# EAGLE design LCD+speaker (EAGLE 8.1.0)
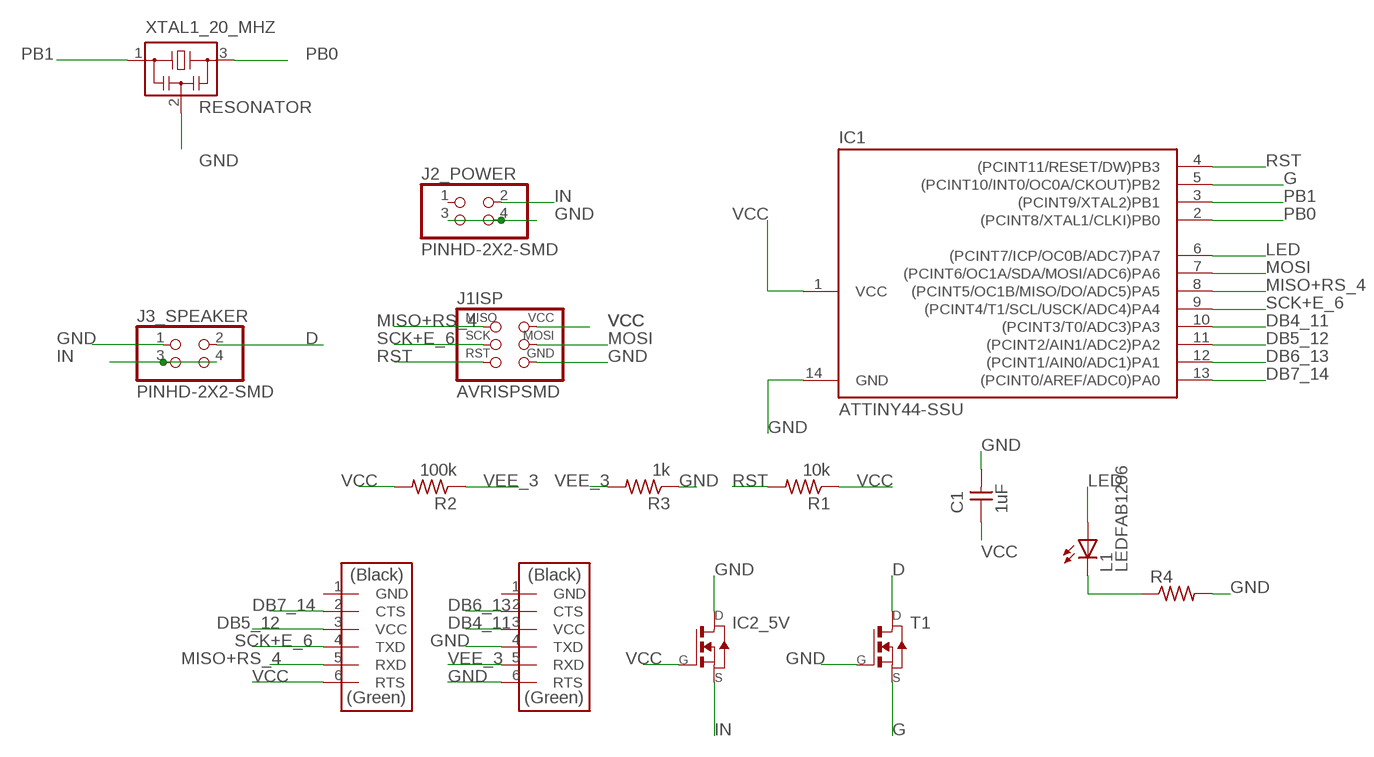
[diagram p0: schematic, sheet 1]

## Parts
C1  1uF  CAP-UNPOLARIZED  [C1206]
IC1  ATTINY44-SSU  [SOIC14]
IC2_5V  NMOSFETSOT23  [SOT-23]
J1ISP  AVRISPSMD  [2X03SMD]
J2_POWER  PINHD-2X2-SMD  [2X02SMD]
J3_SPEAKER  PINHD-2X2-SMD  [2X02SMD]
L1  LEDFAB1206  [LED1206FAB]
R1  10k  RES-US1206FAB  [R1206FAB]
R2  100k  RES-US1206FAB  [R1206FAB]
R3  1k  RES-US1206FAB  [R1206FAB]
R4  RES-US1206FAB  [R1206FAB]
T1  NMOSFETSOT23  [SOT-23]
U$1  FTDI-SMD-HEADER  [1X06SMD]
U$2  FTDI-SMD-HEADER  [1X06SMD]
XTAL1_20_MHZ  RESONATOR  [EFOBM]

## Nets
D: J3_SPEAKER.2 T1.1(D)
DB4_11: IC1.10((PCINT3/T0/ADC3)PA3) U$2.3(VCC)
DB5_12: IC1.11((PCINT2/AIN1/ADC2)PA2) U$1.3(VCC)
DB6_13: IC1.12((PCINT1/AIN0/ADC1)PA1) U$2.2(CTS)
DB7_14: IC1.13((PCINT0/AREF/ADC0)PA0) U$1.2(CTS)
G: IC1.5((PCINT10/INT0/OC0A/CKOUT)PB2) T1.2(S)
GND: C1.2 IC1.14(GND) IC2_5V.1(D) J1ISP.6(GND) J2_POWER.3 J2_POWER.4 J3_SPEAKER.1 R3.1 R4.2 T1.3(G) U$2.4(TXD) U$2.6(RTS) XTAL1_20_MHZ.2
IN: IC2_5V.2(S) J2_POWER.2 J3_SPEAKER.3 J3_SPEAKER.4
LED: IC1.6((PCINT7/ICP/OC0B/ADC7)PA7) L1.1(A)
MISO+RS_4: IC1.8((PCINT5/OC1B/MISO/DO/ADC5)PA5) J1ISP.1(MISO) U$1.5(RXD)
MOSI: IC1.7((PCINT6/OC1A/SDA/MOSI/ADC6)PA6) J1ISP.4(MOSI)
N$3: L1.2(C) R4.1
PB0: IC1.2((PCINT8/XTAL1/CLKI)PB0) XTAL1_20_MHZ.3
PB1: IC1.3((PCINT9/XTAL2)PB1) XTAL1_20_MHZ.1
RST: IC1.4((PCINT11/RESET/DW)PB3) J1ISP.5(RST) R1.2
SCK+E_6: IC1.9((PCINT4/T1/SCL/USCK/ADC4)PA4) J1ISP.3(SCK) U$1.4(TXD)
VCC: C1.1 IC1.1(VCC) IC2_5V.3(G) J1ISP.2(VCC) R1.1 R2.2 U$1.6(RTS)
VEE_3: R2.1 R3.2 U$2.5(RXD)
Unconnected: J2_POWER.1 U$1.1(GND) U$2.1(GND)

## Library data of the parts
C1 = fab:CAP-UNPOLARIZED
IC1 = fab:ATTINY44
IC2_5V T1 = fab:NMOSFET: MOS FET
J1ISP = fab:AVRISP
J2_POWER J3_SPEAKER = fab:PINHD-2X2-SMD
L1 = fab:LED: LED
R1-R4 = fab:RES-US: Resistor (US Symbol)
U$1 U$2 = fab:FTDI-SMD-HEADER
XTAL1_20_MHZ = fab:RESONATOR

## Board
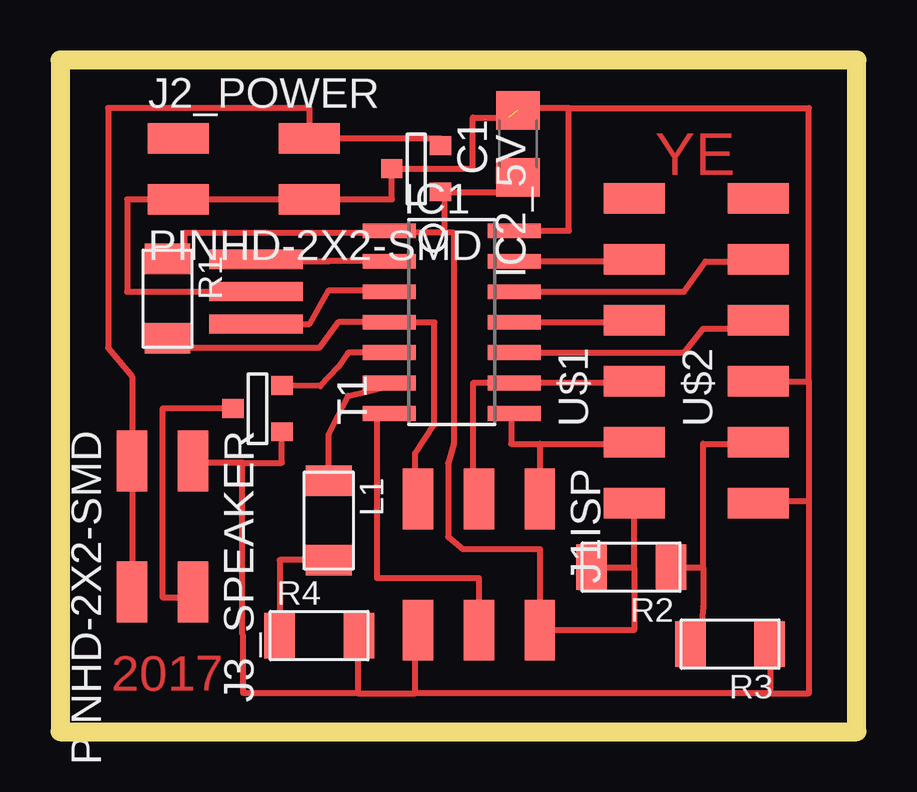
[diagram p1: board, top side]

Size 33.2 x 28 mm. Coordinates in mm from the lower left corner, seen from the top.
Outline: 0,0 33.2,0 33.2,28 0,28 0,0
Copper layers (1*16): Top 0.035mm / dielectric 1.5mm / Bottom 0.035mm
Design rules "default": minimum track width 10mil, minimum drill 24mil, track to track 8mil, track to pad 8mil, pad to pad 8mil, via to via 8mil, smd to smd 8mil, copper to edge 40mil, drill to drill 8mil, minimum pad ring 10mil, minimum via ring 8mil, stop-mask expansion 4mil, vias tented up to drill 0mil, thermal gap 10mil

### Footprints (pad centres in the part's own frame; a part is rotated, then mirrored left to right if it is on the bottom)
C1206 = smd 1.6 x 1.8: 1 -1.4,0; 2 1.4,0
SOIC14 = smd 0.61 x 2.21: 1 -3.81,-2.603; 2 -2.54,-2.603; 3 -1.27,-2.603; 4 0,-2.603; 5 1.27,-2.603; 6 2.54,-2.603; 7 3.81,-2.603; 8 3.81,2.603; 9 2.54,2.603; 10 1.27,2.603; 11 0,2.603; 12 -1.27,2.603; 13 -2.54,2.603; 14 -3.81,2.603
SOT-23 = smd 0.787 x 0.889: 1 0.025,-1.016; 2 -0.94,1.016; 3 0.991,1.016
2X03SMD = smd 2.54 x 1.27: 1 -2.54,2.54; 2 2.92,2.54; 3 -2.54,0; 4 2.92,0; 5 -2.54,-2.54; 6 2.92,-2.54
2X02SMD = smd 2.54 x 1.27: 1 -2.54,1.27; 2 2.92,1.27; 3 -2.54,-1.27; 4 2.92,-1.27
LED1206FAB = smd 1.27 x 1.905: 1 -1.651,0; 2 1.651,0
R1206FAB = smd 1.27 x 1.905: 1 -1.651,0; 2 1.651,0
1X06SMD = smd 2.54 x 1.27: 1 0,6.35; 2 0,3.81; 3 0,1.27; 4 0,-1.27; 5 0,-3.81; 6 0,-6.35
EFOBM = smd 0.8 x 3.9: 1 -1.35,0; 2 0,0; 3 1.35,0

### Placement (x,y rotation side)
C1  19.08,24.5 90 top
IC1  16.33,17.07 270 top
IC2_5V  14.84,23.49 270 top
J1ISP  17.45,7.15 270 top
J2_POWER  7.47,23.45 0 top
J3_SPEAKER  4.27,8.74 270 top
L1  11.2,8.8 270 top
R1  4.48,18.05 270 top
R2  23.8,6.85 180 top
R3  27.92,3.65 180 top
R4  10.8,4 0 top
T1  8.23,13.49 270 top
U$1  23.92,15.87 0 top
U$2  29.1,15.87 0 top
XTAL1_20_MHZ  8.17,18.34 90 top

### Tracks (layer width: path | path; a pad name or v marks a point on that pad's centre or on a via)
D
  Top 0.254: 7.21,13.2 T1.1 4.27,13.46 4.27,5.6 5.54,5.6 J3_SPEAKER.2
DB4_11
  Top 0.254: IC1.10 26,15.8 26.8,16.8 29.1,16.8 U$2.3
DB5_12
  Top 0.254: IC1.11 23.92,17.07 U$1.3
DB6_13
  Top 0.254: IC1.12 26,18.34 26.9,19.6 29.1,19.6 U$2.2
DB7_14
  Top 0.254: IC1.13 23.92,19.61 U$1.2
G
  Top 0.254: 14,15.8 IC1.5 12,15.8 11.6,15.2 10.85,14.4 T1.2
GND  (1 unrouted)
  Top 0.254: XTAL1_20_MHZ.2 2.8,18.34 2.8,22.18 J2_POWER.3 J2_POWER.4 13.82,22.18 IC2_5V.1 17.2,23.46 17.2,25.6 18.68,25.6 | U$2.4 31.2,14.6 | 31.2,14.6 31.2,9.6 | 31.2,9.6 29.1,9.6 U$2.6 | U$2.6 28.4,9.92 | 29.97,4.4 R3.1 | 14.8,1.6 14.8,5.03 J1ISP.6 14.91,4.4 | U$2.6 29.97,9.52 | 31.2,14.6 31.2,26 21.2,26 | 21.2,26 19.08,26 C1.2 | IC1.14 21.2,20.88 21.2,26 | 12.4,1.6 7.65,1.6 7.63,1.62 7.63,4.03 7.6,4.06 7.6,11.2 | 12.4,1.6 14.8,1.6 | 31.2,9.6 31.2,1.6 29.6,1.6 | 29.6,1.6 14.8,1.6 | R3.1 30,4.05 | R3.1 29.6,3.65 29.6,1.6 | R4.2 12.4,4 12.4,1.6 | 7.6,11.2 5.54,11.2 J3_SPEAKER.1 | T1.3 9.25,11.2 7.6,11.2
IN
  Top 0.254: IC2_5V.2 15.86,24.72 J2_POWER.2 10.4,26 2,26 2,16 3,14.8 J3_SPEAKER.3 J3_SPEAKER.4
LED
  Top 0.254: L1.1 11.2,12.4 12,14 13.73,14.4 IC1.6
MISO+RS_4
  Top 0.254: IC1.8 18.8,13.26 18.8,12 19.99,12 | 19.99,12 J1ISP.1 | 19.99,12 23.92,12 U$1.5
MOSI
  Top 0.254: IC1.7 13.2,13.26 13.2,6.4 17.45,6.4 J1ISP.4
N$3
  Top 0.254: L1.2 9.15,7.15 R4.1
PB0
  Top 0.254: 13.73,19.69 IC1.2 11.2,19.61 11.2,19.6 8.17,19.6 XTAL1_20_MHZ.3
PB1
  Top 0.254: XTAL1_20_MHZ.1 10.4,16.99 11.2,18.4 13.73,18.4 IC1.3
RST
  Top 0.254: 13.73,17.2 IC1.4 | IC1.4 15.6,17.07 15.6,12.8 14.8,11.6 14.8,10.49 J1ISP.5 | R1.2 4.4,16.4 4.4,16 10.8,16 11.6,17.07 IC1.4
SCK+E_6
  Top 0.254: U$1.4 23.92,14.53 IC1.9 17.2,14.53 17.2,9.69 J1ISP.3
VCC
  Top 0.254: R1.1 5.2,19.7 5.2,20.8 13.73,20.8 | 16,20.8 16,22.5 IC2_5V.3 19.08,22.5 C1.1 | 16,20.8 13.73,20.8 | 13.73,20.8 IC1.1 | 16,20.8 16.4,20.8 16.4,11.99 16.17,11.19 16.17,8.13 16.8,7.6 19.99,7.6 | 20,7.6 19.99,7.6 | 19.99,7.6 J1ISP.2 23.92,4.23 23.92,6.85 | 23.92,6.85 U$1.6 | R2.2 23.92,6.85
VEE_3
  Top 0.254: R2.1 26.8,6.85 | 26.8,6.85 26.8,12 29.1,12 U$2.5 | R3.2 26.67,4 26.8,5.2 26.8,6.85

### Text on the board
Top: YE | 2017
